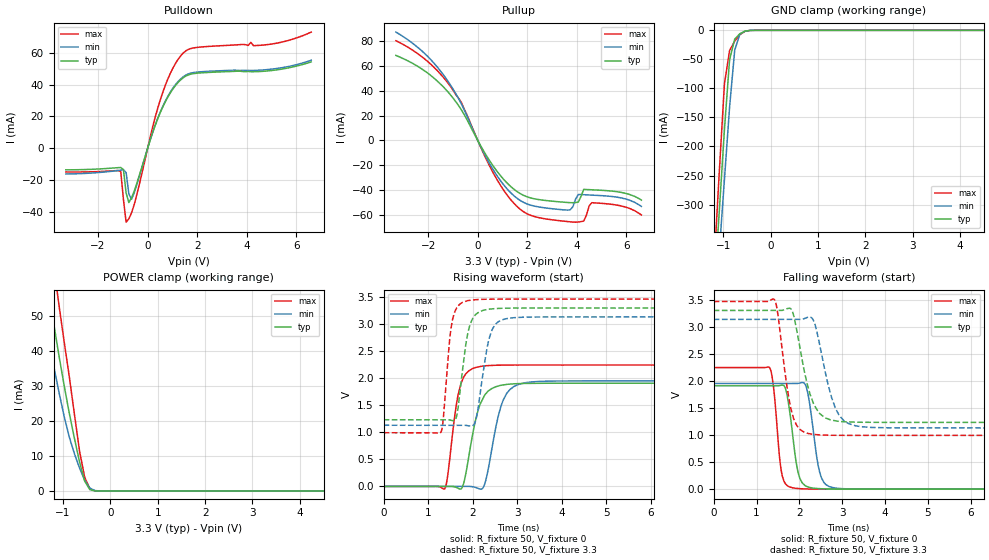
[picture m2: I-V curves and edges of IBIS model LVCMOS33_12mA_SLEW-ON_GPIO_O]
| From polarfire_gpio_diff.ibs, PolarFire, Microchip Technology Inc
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|   Model LVCMOS33_12mA_SLEW-ON_GPIO_O
[Model]   LVCMOS33_12mA_SLEW-ON_GPIO_O
Model_type   Output
Polarity   Non-Inverting
Enable   Active-High
Vmeas =   1.65
Cref =   5p
Rref =   1M
|   typ   min   max
C_comp_pullup   2.605e-12   2.605e-12   2.76e-12
C_comp_pulldown  2.605e-12   2.605e-12   2.76e-12
[Temperature Range]  25C   100C   -40C
[Voltage Range]  3.3   3.135   3.465
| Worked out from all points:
|   slope of the pulldown table from 0 to 0.495 V, typ, clamps not added: 22.7 ohm
|   slope of the pullup table from 0 to 0.495 V, typ, clamps not added: 29.5 ohm
|   GND clamp passes 1 mA (typ) near -0.51 V on its own axis
|   POWER clamp passes 1 mA (typ) near -0.46 V on its own axis
|   rising waveform, R_fixture 50, V_fixture 0: 20-80 % time 293ps typ, 304ps min, 228ps max; typ from 0 V to 1.91 V
|   rising waveform, R_fixture 50, V_fixture 3.3: 20-80 % time 205ps typ, 233ps min, 159ps max; typ from 1.23 V to 3.3 V
|   falling waveform, R_fixture 50, V_fixture 0: 20-80 % time 195ps typ, 210ps min, 149ps max; typ from 1.91 V to 0 V
|   falling waveform, R_fixture 50, V_fixture 3.3: 20-80 % time 350ps typ, 368ps min, 262ps max; typ from 3.3 V to 1.23 V
[GND Clamp]
| Voltage   I(typ)   I(min)   I(max)
-3.3V     -3.213A    -2.957A    -3.541A
-1.191V   -450mA     -505.3mA   -401.1mA
-1.083V   -310.2mA   -380.8mA   -242.7mA
-974.5mV  -170.4mA   -256.4mA   -91.54mA
-866.2mV  -50.48mA   -132.2mA   -34.88mA
-758mV    -15.08mA   -34.24mA   -18.56mA
-649.7mV  -5.883mA   -6.714mA   -7.365mA
-541.4mV  -1.389mA   -1.466mA   -1.709mA
-324.8mV  -3.553uA   -9.504uA   -2.339uA
6.6V      0A         0A         0A
[POWER Clamp]
| Voltage   I(typ)   I(min)   I(max)
-3.3V     320.3mA    266.4mA    379mA
-1.624V   89.11mA    69.3mA     113.8mA
-1.408V   67.23mA    51.37mA    87.82mA
-1.299V   57.08mA    43.14mA    75.67mA
-1.191V   47.51mA    35.38mA    63.94mA
-1.083V   38.51mA    28.09mA    52.96mA
-866.2mV  22.14mA    15.36mA    32.61mA
-649.7mV  8.213mA    6.528mA    11.28mA
-541.4mV  2.791mA    3.019mA    3.88mA
-433.1mV  359.8uA    815.7uA    615.5uA
-216.6mV  159.8nA    4.578uA    2.748uA
6.6V      0A         0A         0A
[Pullup]
| Voltage   I(typ)   I(min)   I(max)
-3.3V     68.42mA    87.18mA    80.23mA
-2.057V   54.76mA    68.39mA    64.18mA
-1.191V   38.81mA    47.31mA    45.9mA
-649.7mV  24.23mA    28.92mA    30.11mA
618.8mV   -20.47mA   -23.48mA   -25.92mA
1.753V    -43.26mA   -48.82mA   -56.06mA
3.733V    -50.12mA   -55.85mA   -65.53mA
4.058V    -49.66mA   -43.55mA   -65.69mA
4.275V    -39.44mA   -43.7mA    -64.96mA
4.599V    -39.74mA   -44.03mA   -50.13mA
5.79V     -41.86mA   -46.3mA    -52.75mA
6.6V      -48.08mA   -53.08mA   -60.03mA
[Pulldown]
| Voltage   I(typ)   I(min)   I(max)
-3.3V     -13.44mA   -16.05mA   -14.79mA
-1.083V   -11.99mA   -13.66mA   -14.59mA
-974.5mV  -13.34mA   -13.38mA   -32.1mA
-866.2mV  -27.94mA   -15.21mA   -46.26mA
-758mV    -33.94mA   -28.44mA   -44.16mA
-649.7mV  -31.06mA   -31.93mA   -40.49mA
515.6mV   22.6mA     22.9mA     30.59mA
928.1mV   35.04mA    35.56mA    47.37mA
1.444V    44.32mA    44.91mA    59.85mA
2.062V    47.18mA    47.87mA    63.37mA
5.141V    49.02mA    49.9mA     65.72mA
6.6V      54.17mA    55.21mA    72.85mA
[Ramp]
dV/dt_r   1.14513/0.293085n  1.17098/0.304325n  1.34717/0.227772n
dV/dt_f   1.2401/0.349781n  1.20209/0.367518n  1.4832/0.262302n
R_load = 50
[Rising Waveform]
R_fixture = 50
V_fixture = 0
V_fixture_min = 0
V_fixture_max = 0
| Time   V(typ)   V(min)   V(max)
0s        49.36nV    35.83nV    137.3nV
1.374ns   841.7uV    662.2uV    -43.44mV
1.637ns   -19.83mV   788.9uV    1.528V
1.736ns   -47.44mV   836.6uV    1.9V
1.832ns   173.1mV    1.021mV    2.064V
2.069ns   1.237V     -19.86mV   2.2V
2.268ns   1.685V     36.59mV    2.229V
2.683ns   1.876V     1.589V     2.243V
3.034ns   1.901V     1.888V     2.245V
10ns      1.909V     1.952V     2.245V
[Rising Waveform]
R_fixture = 50
V_fixture = 3.3
V_fixture_min = 3.135
V_fixture_max = 3.465
| Time   V(typ)   V(min)   V(max)
0s        1.233V     1.132V     993mV
1.289ns   1.233V     1.131V     1.007V
1.34ns    1.233V     1.131V     1.247V
1.551ns   1.217V     1.131V     3.095V
1.657ns   1.365V     1.131V     3.322V
1.88ns    2.786V     1.125V     3.434V
2.077ns   3.185V     1.242V     3.455V
2.381ns   3.279V     2.766V     3.463V
2.686ns   3.295V     3.087V     3.465V
10ns      3.3V       3.135V     3.465V
[Falling Waveform]
R_fixture = 50
V_fixture = 0
V_fixture_min = 0
V_fixture_max = 0
| Time   V(typ)   V(min)   V(max)
0s        1.909V     1.952V     2.245V
1.309ns   1.909V     1.952V     2.237V
1.573ns   1.919V     1.952V     354.2mV
1.702ns   1.777V     1.952V     77.22mV
1.836ns   1.048V     1.952V     25.99mV
1.969ns   307.5mV    1.954V     12.17mV
2.159ns   55mV       1.89V      4.284mV
2.477ns   9.257mV    301.8mV    934.1uV
2.695ns   2.885mV    48.16mV    528.6uV
10ns      602.2nV    3.487uV    255nV
[Falling Waveform]
R_fixture = 50
V_fixture = 3.3
V_fixture_min = 3.135
V_fixture_max = 3.465
| Time   V(typ)   V(min)   V(max)
0s        3.3V       3.135V     3.465V
1.415ns   3.299V     3.135V     3.502V
1.488ns   3.299V     3.134V     3.281V
1.8ns     3.33V      3.134V     1.49V
1.933ns   2.955V     3.134V     1.182V
2.197ns   1.901V     3.176V     1.029V
2.37ns    1.52V      3.026V     1.008V
2.837ns   1.263V     1.502V     994.8mV
3.153ns   1.241V     1.209V     993.4mV
10ns      1.233V     1.132V     993mV
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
